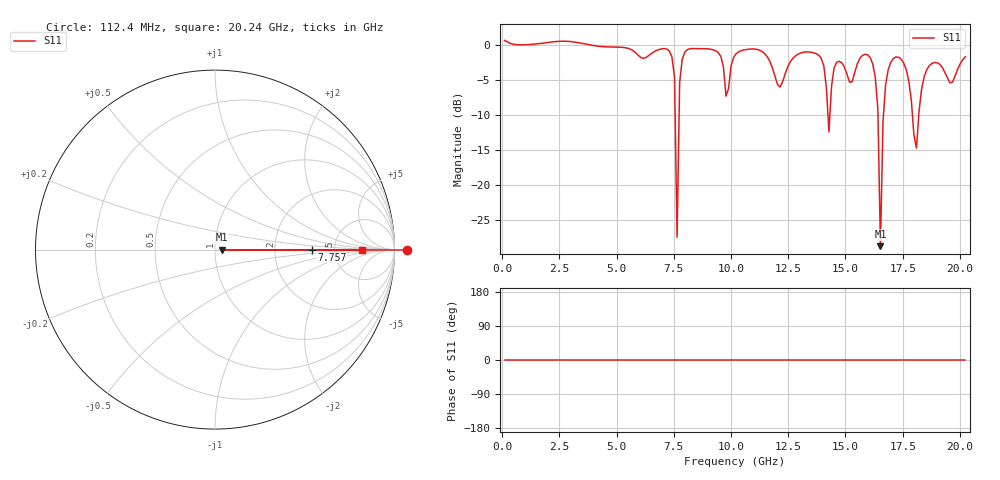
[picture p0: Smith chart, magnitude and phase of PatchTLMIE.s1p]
# GHz S db R 50
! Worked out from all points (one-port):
!   180 points, 112.4 MHz to 20.24 GHz, reference 50 ohm
!   lowest |S11| = -28.7 dB at 16.53 GHz (marker M1), VSWR 1.08, Z = 53.8 + j0 ohm
!   |S11| at or under -10 dB: 7.559 GHz to 7.734 GHz (174.9 MHz wide, 2.29 % of centre); 16.42 GHz to 16.66 GHz (240.9 MHz wide, 1.46 % of centre); 17.92 GHz to 18.2 GHz (279.9 MHz wide, 1.55 % of centre)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
!   S11 on the Smith chart (normalised r, x): 112.4 MHz: -29, -0; 7.757 GHz: 3.33, +0.00; 20.24 GHz: 10, +0
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0.1124222  0.60 0.0
2.698132  0.50 0.0
5.171419  -0.36 0.0
7.419862  -1.75 0.0
7.532284  -4.63 0.0
7.644707  -27.47 0.0
7.757129  -5.38 0.0
8.094395  -0.70 0.0
9.106195  -0.65 0.0
9.780728  -7.34 0.0
10.23042  -1.27 0.0
11.35464  -0.97 0.0
12.14159  -6.05 0.0
12.7037  -1.94 0.0
13.82793  -1.49 0.0
14.27761  -12.46 0.0
14.61488  -2.51 0.0
15.28941  -5.29 0.0
15.85152  -1.36 0.0
16.30121  -4.68 0.0
16.41363  -9.22 0.0
16.52606  -28.75 0.0
16.63848  -10.95 0.0
16.86332  -3.58 0.0
17.7627  -5.15 0.0
18.09997  -14.75 0.0
18.54966  -3.56 0.0
20.23599  -1.72 0.0
